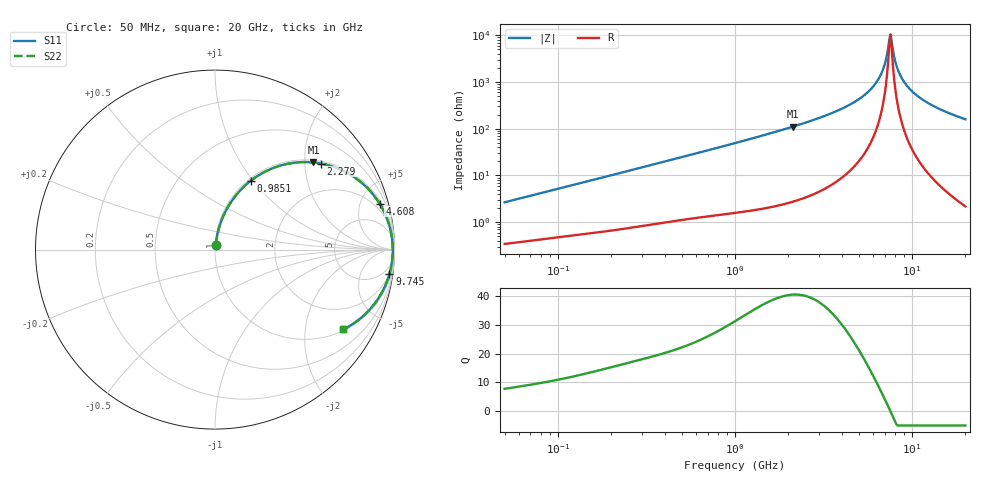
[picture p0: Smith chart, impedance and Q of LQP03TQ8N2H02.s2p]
!Murata Part Number: LQP03TQ8N2H02
!These Parameters are Measured in Series Mode Connection
!  o--[Z]--o
!Port1  Port2
!  o-------o
!Freq. Start=50[MHz] Stop=20[GHz], 401[Steps]
# Hz S RI R 50
!Freq.(Hz) S11(Real) S11(Imag) S21(Real) S21(Imag) S12(Real) S12(Imag) S22(Real) S22(Imag)
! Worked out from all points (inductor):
!   401 points, 50 MHz to 20 GHz, reference 50 ohm
!   read as one part in series: L = 8.32 nH near 51.52 MHz
!   highest Q = 40.5 at 2.115 GHz (marker M1), where L = 8.31 nH
!   self-resonance near 7.442 GHz
!   S11 on the Smith chart (normalised r, x): 50 MHz: 1.01, +0.05; 985.1 MHz: 1.03, +0.97; 2.279 GHz: 1.06, +2.41; 4.608 GHz: 1.28, +7.05; 9.745 GHz: 2, -14; 20 GHz: 1.04, -3.18
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5e7  0.00409 0.0262  0.9959 -0.0262  0.9959 -0.0262  0.00409 0.0262
1.364002e8  0.0101 0.0683  0.9899 -0.0683  0.9899 -0.0683  0.0101 0.0683
3.721004e8  0.0413 0.1751  0.9587 -0.1751  0.9587 -0.1751  0.0413 0.1751
9.85133e8  0.1982 0.3828  0.8018 -0.3828  0.8018 -0.3828  0.1982 0.3828
1e9  0.2028 0.3864  0.7972 -0.3864  0.7972 -0.3864  0.2028 0.3864
2.114743e9  0.5481 0.4855  0.4519 -0.4855  0.4519 -0.4855  0.5481 0.4855
2.279204e9  0.5905 0.4796  0.4095 -0.4796  0.4095 -0.4796  0.5905 0.4796
2.728004e9  0.6902 0.4498  0.3098 -0.4498  0.3098 -0.4498  0.6902 0.4498
3.626126e9  0.8296 0.3613  0.1704 -0.3613  0.1704 -0.3613  0.8296 0.3613
4.608136e9  0.9169 0.2566  0.0831 -0.2566  0.0831 -0.2566  0.9169 0.2566
5.598765e9  0.9634 0.1591  0.0366 -0.1591  0.0366 -0.1591  0.9634 0.1591
6.406762e9  0.9823 0.0879  0.0177 -0.0879  0.0177 -0.0879  0.9823 0.0879
6.905011e9  0.988 0.0477  0.012 -0.0477  0.012 -0.0477  0.988 0.0477
7.442007e9  0.9905 0.00714  0.00953 -0.00714  0.00953 -0.00714  0.9905 0.00714
7.668323e9  0.9905 -0.00909  0.00949 0.00909  0.00949 0.00909  0.9905 -0.00909
8.141811e9  0.989 -0.0415  0.011 0.0415  0.011 0.0415  0.989 -0.0415
8.516016e9  0.9864 -0.0658  0.0136 0.0658  0.0136 0.0658  0.9864 -0.0658
9.041845e9  0.9811 -0.098  0.0189 0.098  0.0189 0.098  0.9811 -0.098
9.745021e9  0.9714 -0.1379  0.0286 0.1379  0.0286 0.1379  0.9714 -0.1379
1.098561e10  0.9489 -0.2001  0.0511 0.2001  0.0511 0.2001  0.9489 -0.2001
1.295331e10  0.9039 -0.2811  0.0961 0.2811  0.0961 0.2811  0.9039 -0.2811
2e10  0.7142 -0.445  0.2858 0.445  0.2858 0.445  0.7142 -0.445
